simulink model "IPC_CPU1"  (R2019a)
settings: Solver=FixedStepDiscrete  StartTime=0.0  StopTime=2  RelTol=1e-3  EnableMultiTasking=on
libraries: c2837xDlib x1

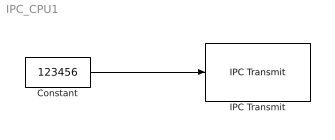
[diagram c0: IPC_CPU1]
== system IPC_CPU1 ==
  Constant : Constant  Value=123456  VectorParams1D=off  OutDataTypeStr=uint32  SampleTime=0.5
  IPC Transmit : c2837xDlib/IPC Transmit  SelectChannel=24  EnableBlocking=off
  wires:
  Constant/1 -> IPC Transmit/1
